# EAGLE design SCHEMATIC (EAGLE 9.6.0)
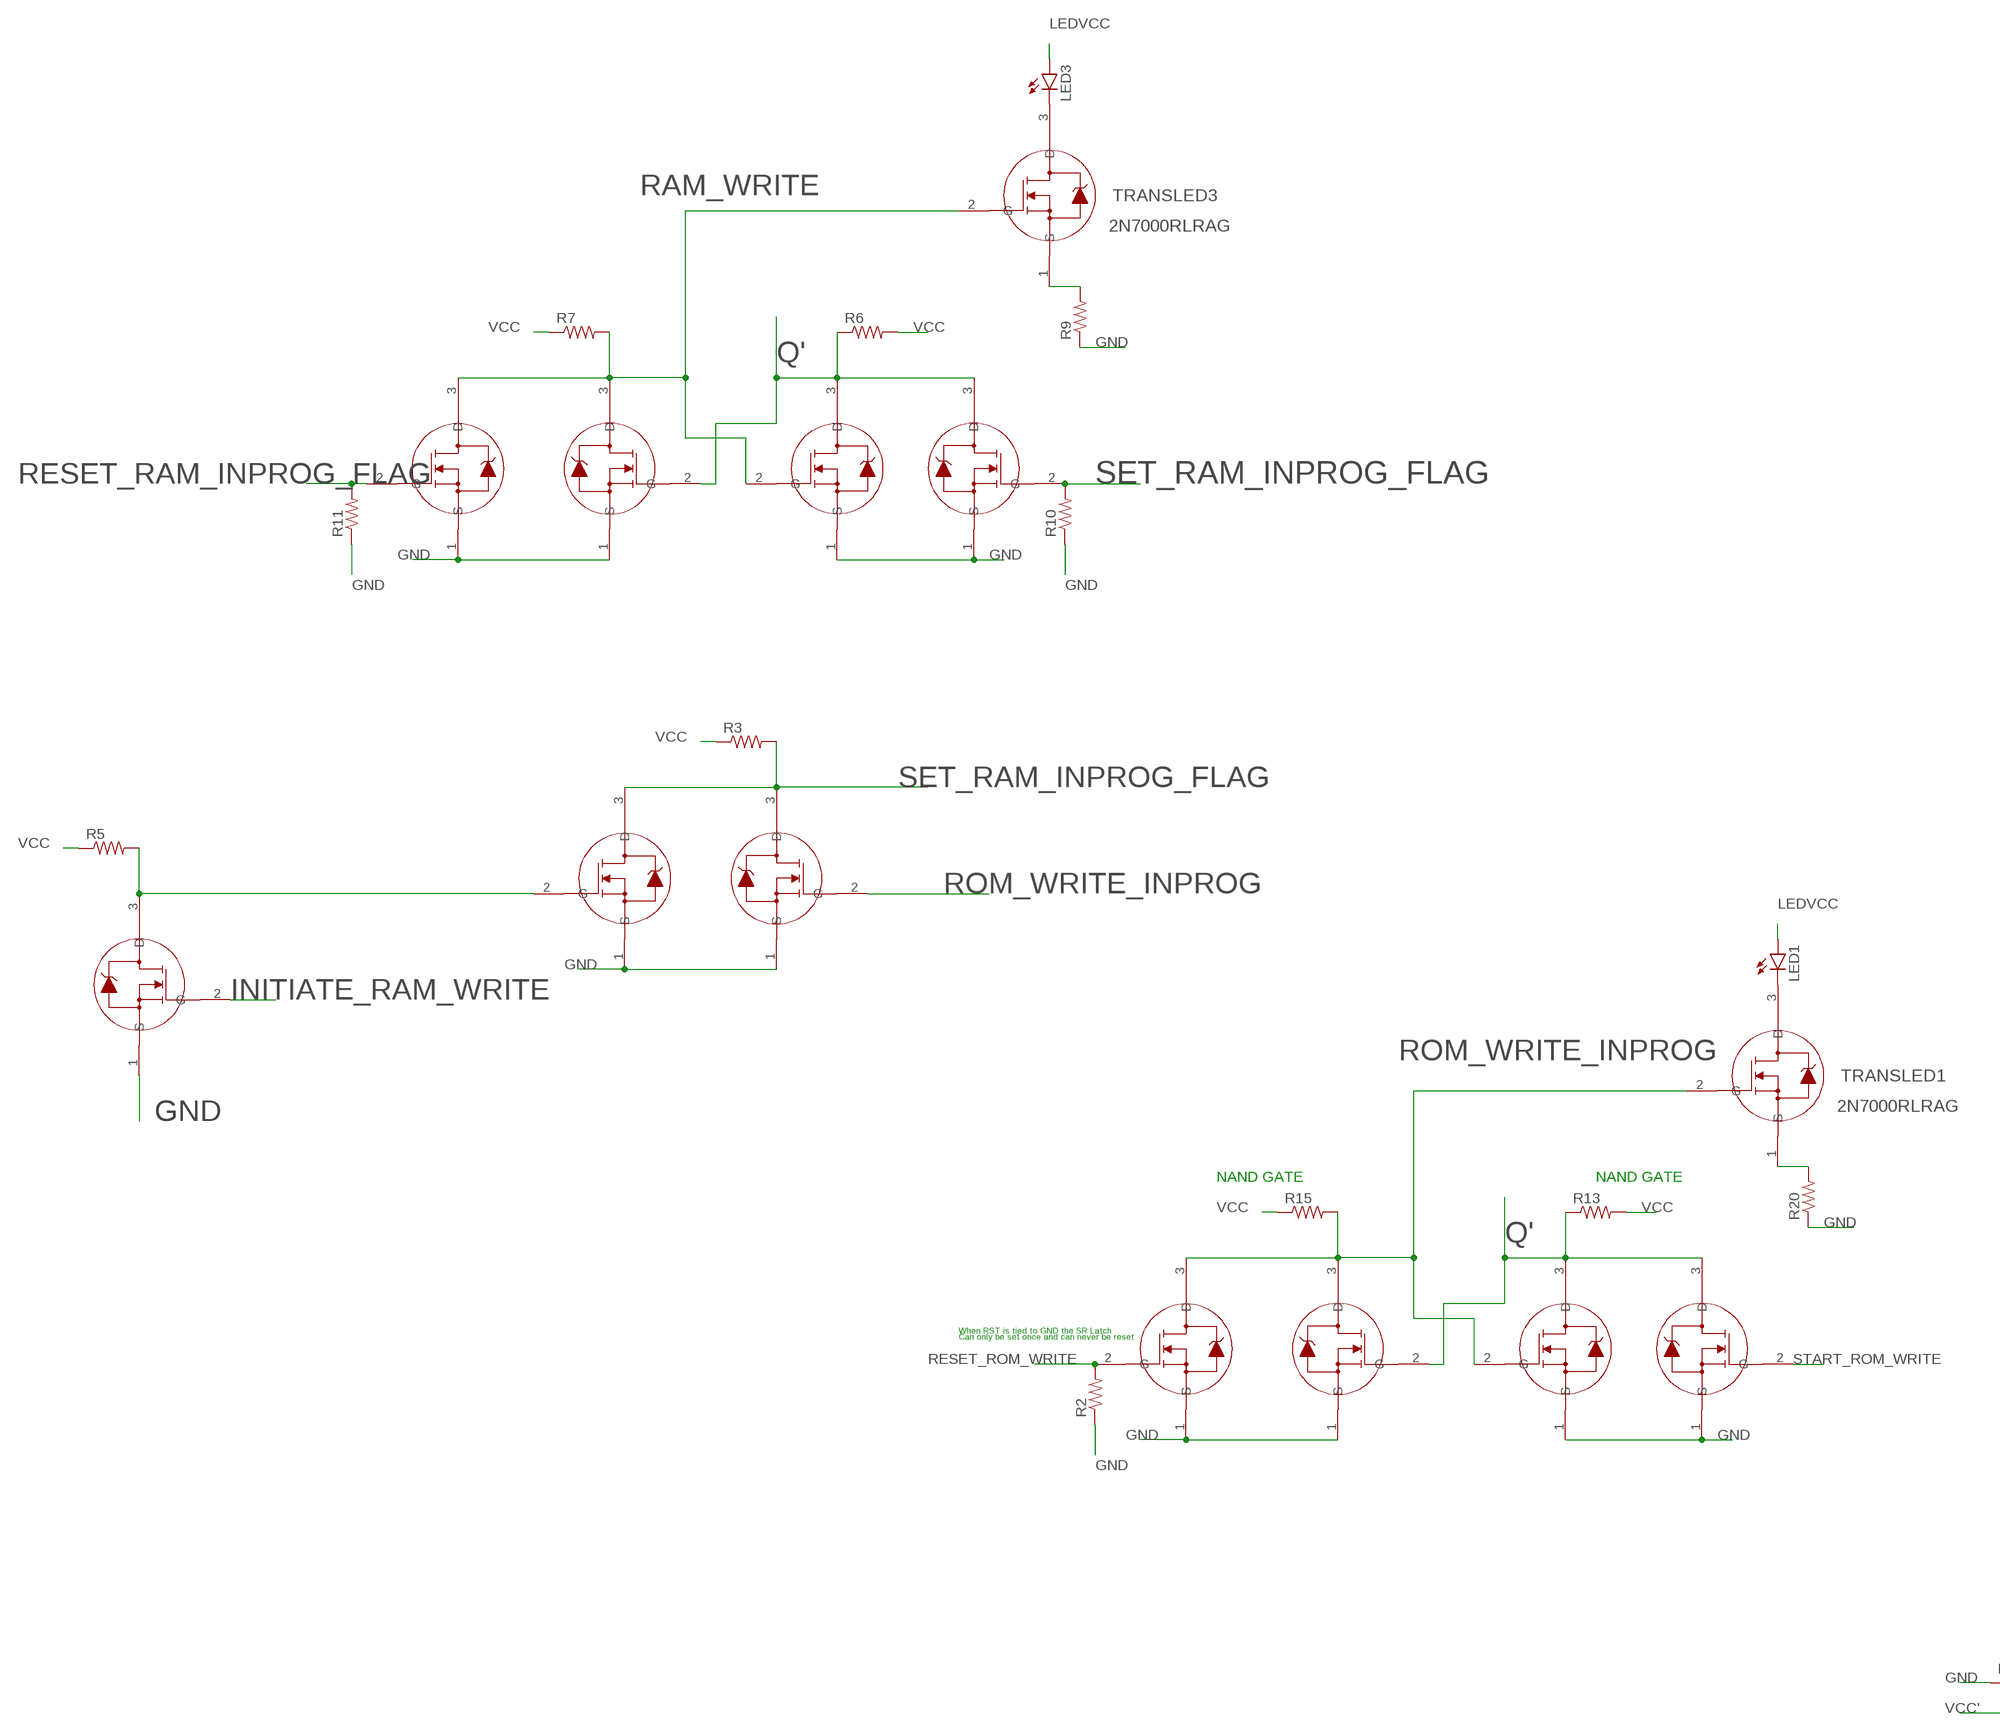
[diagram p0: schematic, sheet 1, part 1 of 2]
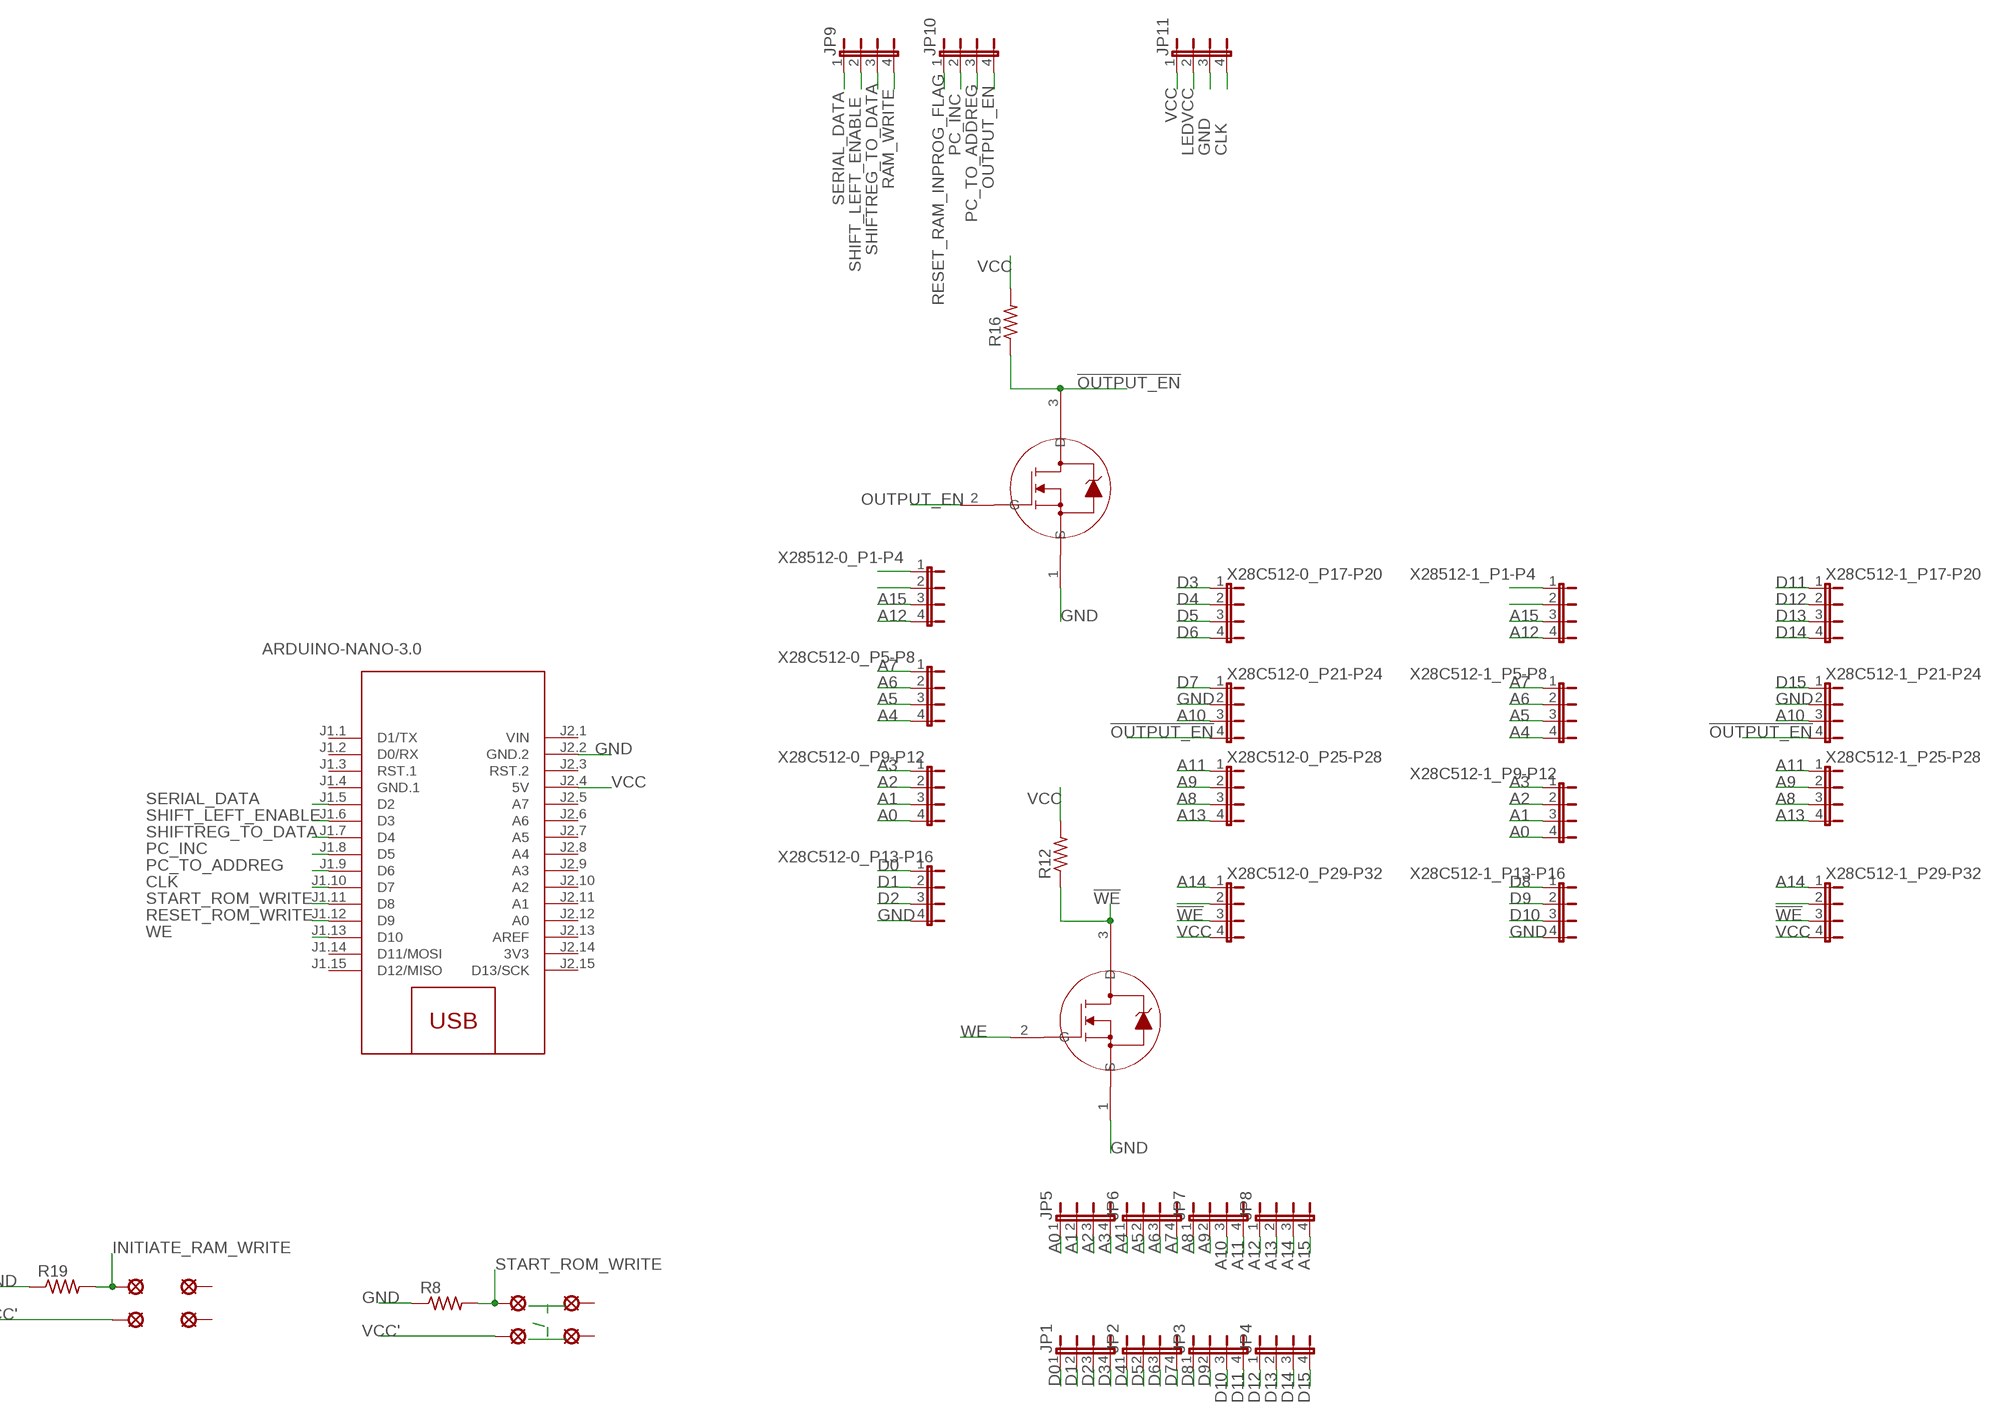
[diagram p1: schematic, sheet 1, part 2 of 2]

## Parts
B1_BL  SE14  [SE14]
B1_BL3  SE14  [SE14]
B1_BR  SE14  [SE14]
B1_BR3  SE14  [SE14]
B1_TL  SE14  [SE14]
B1_TL3  SE14  [SE14]
B1_TR  SE14  [SE14]
B1_TR3  SE14  [SE14]
JP1  JP4E  [JP4]
JP2  JP4E  [JP4]
JP3  JP4E  [JP4]
JP4  JP4E  [JP4]
JP5  JP4E  [JP4]
JP6  JP4E  [JP4]
JP7  JP4E  [JP4]
JP8  JP4E  [JP4]
JP9  JP4E  [JP4]
JP10  JP4E  [JP4]
JP11  JP4E  [JP4]
LED1  LED3MM  [LED3MM]
LED3  LED3MM  [LED3MM]
M1  ARDUINO-NANO-3.0  [ARDUINO-NANO-3.0]
NFET1  2N7000RLRAG  [TO-92_ONS]
NFET2  2N7000RLRAG  [TO-92_ONS]
NFET3  2N7000RLRAG  [TO-92_ONS]
NFET4  2N7000RLRAG  [TO-92_ONS]
NFET5  2N7000RLRAG  [TO-92_ONS]
NFET6  2N7000RLRAG  [TO-92_ONS]
NFET7  2N7000RLRAG  [TO-92_ONS]
NFET8  2N7000RLRAG  [TO-92_ONS]
NFET10  2N7000RLRAG  [TO-92_ONS]
NFET19  2N7000RLRAG  [TO-92_ONS]
NFET20  2N7000RLRAG  [TO-92_ONS]
NFET21  2N7000RLRAG  [TO-92_ONS]
NFET22  2N7000RLRAG  [TO-92_ONS]
R2  R-US_0204/7  [0204/7]
R3  R-US_0204/7  [0204/7]
R5  R-US_0204/7  [0204/7]
R6  R-US_0204/7  [0204/7]
R7  R-US_0204/7  [0204/7]
R8  R-US_0204/7  [0204/7]
R9  R-US_0204/7  [0204/7]
R10  R-US_0204/7  [0204/7]
R11  R-US_0204/7  [0204/7]
R12  R-US_0204/7  [0204/7]
R13  R-US_0204/7  [0204/7]
R15  R-US_0204/7  [0204/7]
R16  R-US_0204/7  [0204/7]
R19  R-US_0204/7  [0204/7]
R20  R-US_0204/7  [0204/7]
TRANSLED1  2N7000RLRAG  [TO-92_ONS]
TRANSLED3  2N7000RLRAG  [TO-92_ONS]
X28C512-0_P5-P8  JP4E  [JP4]
X28C512-0_P9-P12  JP4E  [JP4]
X28C512-0_P13-P16  JP4E  [JP4]
X28C512-0_P17-P20  JP4E  [JP4]
X28C512-0_P21-P24  JP4E  [JP4]
X28C512-0_P25-P28  JP4E  [JP4]
X28C512-0_P29-P32  JP4E  [JP4]
X28C512-1_P5-P8  JP4E  [JP4]
X28C512-1_P9-P12  JP4E  [JP4]
X28C512-1_P13-P16  JP4E  [JP4]
X28C512-1_P17-P20  JP4E  [JP4]
X28C512-1_P21-P24  JP4E  [JP4]
X28C512-1_P25-P28  JP4E  [JP4]
X28C512-1_P29-P32  JP4E  [JP4]
X28512-0_P1-P4  JP4E  [JP4]
X28512-1_P1-P4  JP4E  [JP4]

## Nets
!OUTPUT_EN: NFET10.3(D) R16.1 X28C512-0_P21-P24.4 X28C512-1_P21-P24.4
!WE: NFET4.3(D) R12.1 X28C512-0_P29-P32.3 X28C512-1_P29-P32.3
A0: JP5.1 X28C512-0_P9-P12.4 X28C512-1_P9-P12.4
A1: JP5.2 X28C512-0_P9-P12.3 X28C512-1_P9-P12.3
A2: JP5.3 X28C512-0_P9-P12.2 X28C512-1_P9-P12.2
A3: JP5.4 X28C512-0_P9-P12.1 X28C512-1_P9-P12.1
A4: JP6.1 X28C512-0_P5-P8.4 X28C512-1_P5-P8.4
A5: JP6.2 X28C512-0_P5-P8.3 X28C512-1_P5-P8.3
A6: JP6.3 X28C512-0_P5-P8.2 X28C512-1_P5-P8.2
A7: JP6.4 X28C512-0_P5-P8.1 X28C512-1_P5-P8.1
A8: JP7.1 X28C512-0_P25-P28.3 X28C512-1_P25-P28.3
A9: JP7.2 X28C512-0_P25-P28.2 X28C512-1_P25-P28.2
A10: JP7.3 X28C512-0_P21-P24.3 X28C512-1_P21-P24.3
A11: JP7.4 X28C512-0_P25-P28.1 X28C512-1_P25-P28.1
A12: JP8.1 X28512-0_P1-P4.4 X28512-1_P1-P4.4
A13: JP8.2 X28C512-0_P25-P28.4 X28C512-1_P25-P28.4
A14: JP8.3 X28C512-0_P29-P32.1 X28C512-1_P29-P32.1
A15: JP8.4 X28512-0_P1-P4.3 X28512-1_P1-P4.3
CLK: JP11.4 M1.J1.10(D7)
D0: JP1.1 X28C512-0_P13-P16.1
D1: JP1.2 X28C512-0_P13-P16.2
D2: JP1.3 X28C512-0_P13-P16.3
D3: JP1.4 X28C512-0_P17-P20.1
D4: JP2.1 X28C512-0_P17-P20.2
D5: JP2.2 X28C512-0_P17-P20.3
D6: JP2.3 X28C512-0_P17-P20.4
D7: JP2.4 X28C512-0_P21-P24.1
D8: JP3.1 X28C512-1_P13-P16.1
D9: JP3.2 X28C512-1_P13-P16.2
D10: JP3.3 X28C512-1_P13-P16.3
D11: JP3.4 X28C512-1_P17-P20.1
D12: JP4.1 X28C512-1_P17-P20.2
D13: JP4.2 X28C512-1_P17-P20.3
D14: JP4.3 X28C512-1_P17-P20.4
D15: JP4.4 X28C512-1_P21-P24.1
GND: JP11.3 M1.J2.2(GND.2) NFET1.1(S) NFET2.1(S) NFET3.1(S) NFET4.1(S) NFET5.1(S) NFET6.1(S) NFET7.1(S) NFET8.1(S) NFET10.1(S) NFET19.1(S) NFET20.1(S) NFET21.1(S) NFET22.1(S) R2.1 R8.1 R9.1 R10.1 R11.1 R19.1 R20.1 X28C512-0_P13-P16.4 X28C512-0_P21-P24.2 X28C512-1_P13-P16.4 X28C512-1_P21-P24.2
INITIATE_RAM_WRITE: B1_TL3.MP NFET3.2(G) R19.2
LEDVCC: JP11.2 LED1.A LED3.A
N$1: X28512-0_P1-P4.1
N$2: X28512-0_P1-P4.2
N$5: LED3.K(C) TRANSLED3.3(D)
N$6: R9.2 TRANSLED3.1(S)
N$17: X28512-1_P1-P4.1
N$18: X28512-1_P1-P4.2
N$22: X28C512-0_P29-P32.2
N$41: LED1.K(C) TRANSLED1.3(D)
N$42: R20.2 TRANSLED1.1(S)
N$44: X28C512-1_P29-P32.2
OUTPUT_EN: JP10.4 NFET10.2(G)
PC_INC: JP10.2 M1.J1.8(D5)
PC_TO_ADDREG: JP10.3 M1.J1.9(D6)
Q': NFET5.2(G) NFET7.3(D) NFET8.3(D) NFET19.2(G) NFET21.3(D) NFET22.3(D) R6.1 R13.1
RAM_WRITE: JP9.4 NFET5.3(D) NFET6.3(D) NFET7.2(G) R7.2 TRANSLED3.2(G)
RAM_WRITE_FLAG: NFET2.2(G) NFET3.3(D) R5.2
RESET_RAM_INPROG_FLAG: JP10.1 NFET6.2(G) R11.2
RESET_ROM_WRITE: M1.J1.12(D9) NFET20.2(G) R2.2
ROM_WRITE_INPROG: NFET1.2(G) NFET19.3(D) NFET20.3(D) NFET21.2(G) R15.2 TRANSLED1.2(G)
SERIAL_DATA: JP9.1 M1.J1.5(D2)
SET_RAM_INPROG_FLAG: NFET1.3(D) NFET2.3(D) NFET8.2(G) R3.2 R10.2
SHIFT_LEFT_ENABLE: JP9.2 M1.J1.6(D3)
SHIFTREG_TO_DATA: JP9.3 M1.J1.7(D4)
START_ROM_WRITE: B1_TL.MP M1.J1.11(D8) NFET22.2(G) R8.2
VCC: JP11.1 M1.J2.4(5V) R3.1 R5.1 R6.2 R7.1 R12.2 R13.2 R15.1 R16.2 X28C512-0_P29-P32.4 X28C512-1_P29-P32.4
VCC': B1_BL3.MP B1_BL.MP
WE: M1.J1.13(D10) NFET4.2(G)
Unconnected: B1_BR3.MP B1_BR.MP B1_TR3.MP B1_TR.MP M1.J1.1(D1/TX) M1.J1.2(D0/RX) M1.J1.3(RST.1) M1.J1.14(D11/MOSI) M1.J1.15(D12/MISO) M1.J2.3(RST.2) M1.J2.5(A7) M1.J2.6(A6) M1.J2.7(A5) M1.J2.8(A4) M1.J2.9(A3) M1.J2.10(A2) M1.J2.11(A1) M1.J2.12(A0) M1.J2.13(AREF) M1.J2.15(D13/SCK)

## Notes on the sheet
- NAND GATE | NAND GATE
- Can only be set once and can never be reset | When RST is tied to GND the SR Latch
- ____
- ____ | _ | _/  _

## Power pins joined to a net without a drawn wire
3V3: M1.J2.14(3V3)
GND.1: M1.J1.4(GND.1)
VIN: M1.J2.1(VIN)

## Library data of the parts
B1_BL B1_BL3 B1_BR B1_BR3 B1_TL B1_TL3 B1_TR B1_TR3 = solpad:SE14: SOLDER PAD
JP1-JP11 X28C512-0_P5-P8 X28C512-0_P9-P12 X28C512-0_P13-P16 X28C512-0_P17-P20 X28C512-0_P21-P24 X28C512-0_P25-P28 X28C512-0_P29-P32 X28C512-1_P5-P8 X28C512-1_P9-P12 X28C512-1_P13-P16 X28C512-1_P17-P20 X28C512-1_P21-P24 X28C512-1_P25-P28 X28C512-1_P29-P32 X28512-0_P1-P4 X28512-1_P1-P4 = jumper:JP4E: JUMPER
LED1 LED3 = led:LED: LED
M1 = JD-WEEK_8_9_1:ARDUINO-NANO-3.0: Arduino Nano 3.0 and compatible devices More details available here: https://www.arduino.cc/en/Main/ArduinoBoardNano Click here to find device on ebay.com
NFET1-NFET8 NFET10 NFET19-NFET22 TRANSLED1 TRANSLED3 = Transistor(MOSFET):2N7000RLRAG; COPYRIGHT: Copyright (C) 2022 Ultra Librarian. All rights reserved.; MANUFACTURER_PART_NUMBER: 2N7000RLRAG; MFR_NAME: onsemi
R2 R3 R5-R13 R15 R16 R19 R20 = rcl:R-US_: RESISTOR, American symbol; SPICEPREFIX: R

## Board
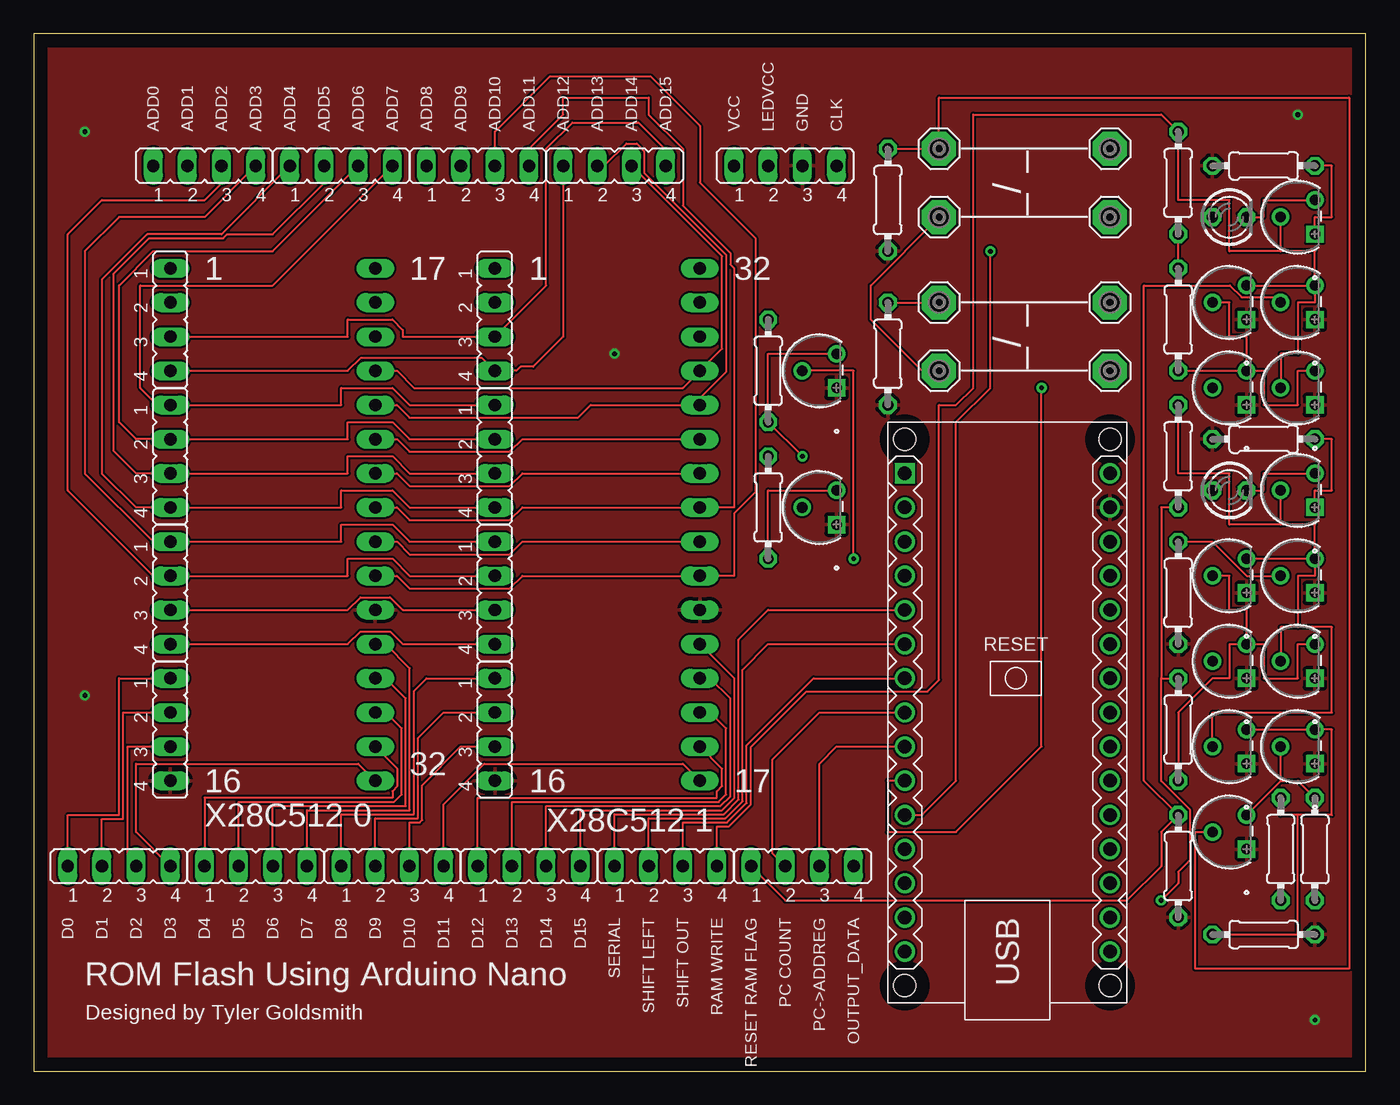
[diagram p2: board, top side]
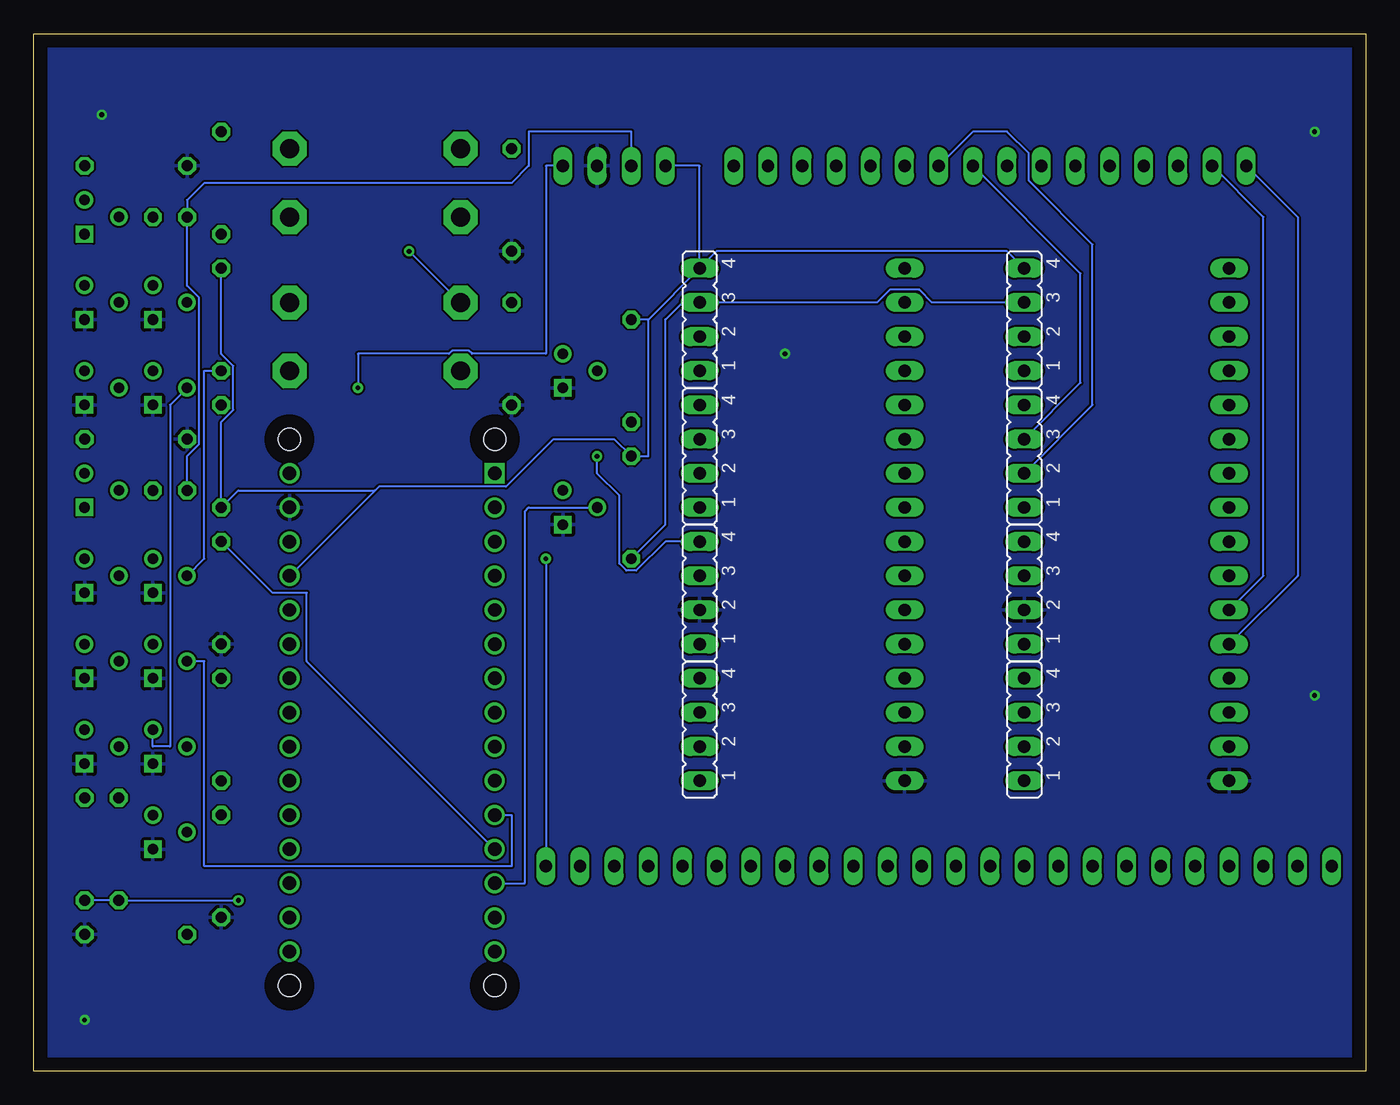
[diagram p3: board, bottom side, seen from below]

Size 99.04 x 77.14 mm. Coordinates in mm from the lower left corner, seen from the top.
Outline: 0,0 99.04,0 99.04,77.14 0,77.14 0,0
Copper layers (1*16): Top 0.035mm / dielectric 1.5mm / Bottom 0.035mm
Design rules "default *": minimum track width 6mil, minimum drill 0.35mm, track to track 6mil, track to pad 6mil, pad to pad 6mil, via to via 6mil, smd to smd 6mil, copper to edge 40mil, drill to drill 6mil, minimum pad ring 10mil, minimum via ring 8mil, stop-mask expansion 4mil, vias tented up to drill 0mil, thermal gap 10mil

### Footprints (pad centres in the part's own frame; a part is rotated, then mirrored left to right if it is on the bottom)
SE14 = drill 1.397 pad 2.54 octagon: MP 0,0
JP4 = drill 0.914 long: 1 -3.81,0; 2 -1.27,0; 3 1.27,0; 4 3.81,0
LED3MM = drill 0.813 octagon: A -1.27,0; K 1.27,0
ARDUINO-NANO-3.0 = drill 1 square: J1.1 17.78,7.62 | drill 1: J1.2 15.24,7.62; J1.3 12.7,7.62; J1.4 10.16,7.62; J1.5 7.62,7.62; J1.6 5.08,7.62; J1.7 2.54,7.62; J1.8 0,7.62; J1.9 -2.54,7.62; J1.10 -5.08,7.62; J1.11 -7.62,7.62; J1.12 -10.16,7.62; J1.13 -12.7,7.62; J1.14 -15.24,7.62; J1.15 -17.78,7.62; J2.1 17.78,-7.62; J2.2 15.24,-7.62; J2.3 12.7,-7.62; J2.4 10.16,-7.62; J2.5 7.62,-7.62; J2.6 5.08,-7.62; J2.7 2.54,-7.62; J2.8 0,-7.62; J2.9 -2.54,-7.62; J2.10 -5.08,-7.62; J2.11 -7.62,-7.62; J2.12 -10.16,-7.62; J2.13 -12.7,-7.62; J2.14 -15.24,-7.62; J2.15 -17.78,-7.62 | hole 1.651: -20.32,7.62; -20.32,-7.62; 20.32,-7.62; 20.32,7.62
TO-92_ONS = drill 0.787 pad 1.295 square: 1 0,0 | drill 0.787 pad 1.295: 2 1.27,2.54; 3 2.54,0
0204/7 = drill 0.813 octagon: 1 -3.81,0; 2 3.81,0

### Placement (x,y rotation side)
B1_BL  67.31,52.07 0 top
B1_BL3  67.31,63.5 0 top
B1_BR  80.01,52.07 0 top
B1_BR3  80.01,63.5 0 top
B1_TL  67.31,57.15 0 top
B1_TL3  67.31,68.58 0 top
B1_TR  80.01,57.15 0 top
B1_TR3  80.01,68.58 0 top
JP1  6.35,15.24 0 top
JP2  16.51,15.24 0 top
JP3  26.67,15.24 0 top
JP4  36.83,15.24 0 top
JP5  12.7,67.31 0 top
JP6  22.86,67.31 0 top
JP7  33.02,67.31 0 top
JP8  43.18,67.31 0 top
JP9  46.99,15.24 0 top
JP10  57.15,15.24 0 top
JP11  55.88,67.31 0 top
LED1  88.9,43.18 0 top
LED3  88.9,63.5 0 top
M1  72.39,26.67 90 top
NFET1  90.17,22.86 90 top
NFET2  95.25,22.86 90 top
NFET3  90.17,16.51 90 top
NFET4  59.69,40.64 90 top
NFET5  90.17,55.88 90 top
NFET6  95.25,55.88 90 top
NFET7  95.25,49.53 90 top
NFET8  90.17,49.53 90 top
NFET10  59.69,50.8 90 top
NFET19  90.17,35.56 90 top
NFET20  95.25,35.56 90 top
NFET21  95.25,29.21 90 top
NFET22  90.17,29.21 90 top
R2  85.09,35.56 90 top
R3  92.71,16.51 90 top
R5  95.25,16.51 90 top
R6  85.09,55.88 90 top
R7  85.09,66.04 90 top
R8  63.5,53.34 90 top
R9  91.44,67.31 0 top
R10  91.44,10.16 180 top
R11  85.09,15.24 90 top
R12  54.61,41.91 90 top
R13  85.09,25.4 90 top
R15  85.09,45.72 90 top
R16  54.61,52.07 90 top
R19  63.5,64.77 90 top
R20  91.44,46.99 0 top
TRANSLED1  95.25,41.91 90 top
TRANSLED3  95.25,62.23 90 top
X28C512-0_P5-P8  10.16,45.72 270 top
X28C512-0_P9-P12  10.16,35.56 270 top
X28C512-0_P13-P16  10.16,25.4 270 top
X28C512-0_P17-P20  25.4,25.4 90 bottom
X28C512-0_P21-P24  25.4,35.56 90 bottom
X28C512-0_P25-P28  25.4,45.72 90 bottom
X28C512-0_P29-P32  25.4,55.88 90 bottom
X28C512-1_P5-P8  34.29,45.72 270 top
X28C512-1_P9-P12  34.29,35.56 270 top
X28C512-1_P13-P16  34.29,25.4 270 top
X28C512-1_P17-P20  49.53,25.4 90 bottom
X28C512-1_P21-P24  49.53,35.56 90 bottom
X28C512-1_P25-P28  49.53,45.72 90 bottom
X28C512-1_P29-P32  49.53,55.88 90 bottom
X28512-0_P1-P4  10.16,55.88 270 top
X28512-1_P1-P4  34.29,55.88 270 top

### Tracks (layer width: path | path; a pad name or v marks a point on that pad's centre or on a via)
!OUTPUT_EN  (via drill 0.35)
  Top 0.152: X28C512-0_P21-P24.4 27.01,39.37 27.95,38.43 35.39,38.43 36.33,39.37 X28C512-1_P21-P24.4 | NFET10.3 54.61,53.34 R16.1 v57.15,45.72
  Bottom 0.152: v57.15,45.72 57.15,44.45 55.5,42.8 55.5,37.73 54.98,37.21 54.24,37.21 52.08,39.37 X28C512-1_P21-P24.4
!WE
  Top 0.152: R12.1 54.61,43.18 NFET4.3
  Bottom 0.152: R12.1 52.07,40.64 52.07,55.88 50.8,57.15 X28C512-1_P29-P32.3 36.33,57.15 35.39,58.09 33.19,58.09 32.25,57.15 X28C512-0_P29-P32.3
A0
  Top 0.152: X28C512-0_P9-P12.4 23.36,31.75 24.3,32.69 26.5,32.69 27.44,31.75 X28C512-1_P9-P12.4
  Bottom 0.152: JP5.1 5.08,63.5 5.08,36.83 X28C512-0_P9-P12.4
A1
  Top 0.152: X28C512-0_P9-P12.3 23.36,34.29 24.3,35.23 26.5,35.23 27.44,34.29 X28C512-1_P9-P12.3
  Bottom 0.152: X28C512-0_P9-P12.3 7.62,36.83 7.62,63.5 JP5.2
A2
  Top 0.152: JP5.3 13.97,66.04 12.7,64.77 5.08,64.77 2.54,62.23 2.54,43.18 8.89,36.83 X28C512-0_P9-P12.2 23.36,36.83 23.36,38.1 26.67,38.1 27.94,36.83 X28C512-1_P9-P12.2
A3
  Top 0.152: JP5.4 12.7,63.5 6.35,63.5 3.81,60.96 3.81,44.45 8.89,39.37 X28C512-0_P9-P12.1 22.86,39.37 22.86,40.64 26.67,40.64 27.94,39.37 X28C512-1_P9-P12.1
A4
  Top 0.152: JP6.1 13.97,62.23 8.46,62.23 5.08,58.85 5.08,44.45 7.62,41.91 X28C512-0_P5-P8.4 22.86,41.91 22.86,43.18 26.67,43.18 27.94,41.91 X28C512-1_P5-P8.4
A5
  Top 0.152: JP6.2 21.59,66.04 17.78,62.23 14.4,62.23 14.1,61.92 8.59,61.92 5.97,59.31 5.97,46.1 7.62,44.45 X28C512-0_P5-P8.3 23.36,44.45 23.36,45.72 26.67,45.72 27.94,44.45 X28C512-1_P5-P8.3
A6
  Top 0.152: JP6.3 17.78,60.96 8.89,60.96 6.35,58.42 6.35,48.26 7.62,46.99 X28C512-0_P5-P8.2 23.36,46.99 23.36,48.26 26.67,48.26 27.94,46.99 X28C512-1_P5-P8.2
A7
  Top 0.152: JP6.4 17.78,58.42 7.92,58.42 7.92,50.8 9.2,49.53 X28C512-0_P5-P8.1 22.86,49.53 22.86,50.8 26.67,50.8 27.94,49.53 X28C512-1_P5-P8.1
A8
  Top 0.152: X28C512-0_P25-P28.3 27.01,46.99 27.95,46.05 35.39,46.05 36.33,46.99 X28C512-1_P25-P28.3
  Bottom 0.152: JP7.1 21.21,59.31 21.21,51.18 X28C512-0_P25-P28.3
A9
  Top 0.152: X28C512-0_P25-P28.2 27.01,44.45 27.95,43.51 35.39,43.51 36.33,44.45 X28C512-1_P25-P28.2
  Bottom 0.152: X28C512-0_P25-P28.2 20.32,49.53 20.32,61.46 25.07,66.21 25.07,68.25 26.67,69.85 29.21,69.85 JP7.2
A10
  Top 0.152: X28C512-0_P21-P24.3 27.01,36.83 27.95,35.89 35.39,35.89 36.33,36.83 X28C512-1_P21-P24.3 52.07,36.83 52.07,41.48 53.64,43.05 53.64,61.95 49.53,66.06 49.53,70.28 45.85,73.97 38.41,73.97 34.29,69.85 JP7.3
A11
  Top 0.152: X28C512-0_P25-P28.1 27.01,41.91 27.95,40.97 35.39,40.97 36.33,41.91 X28C512-1_P25-P28.1 52.07,41.91 52.07,59.69 51.79,59.97 51.79,60.83 48.26,64.36 48.26,68.58 45.72,71.12 45.72,72.39 39.37,72.39 39.37,71.12 36.83,68.58 JP7.4
A12
  Top 0.152: X28512-0_P1-P4.4 23.36,52.07 24.3,53.01 33.35,53.01 X28512-1_P1-P4.4 35.9,52.07 36.2,52.38 37.14,52.38 39.37,54.61 JP8.1
A13
  Top 0.152: X28C512-0_P25-P28.4 27.01,49.53 27.95,48.59 40.47,48.59 41.41,49.53 X28C512-1_P25-P28.4 49.53,50.03 51.49,51.99 51.49,60.7 45.39,66.8 45.39,68.41 44.84,68.96 44.06,68.96 42.41,67.31 JP8.2
A14
  Top 0.152: X28C512-0_P29-P32.1 27.01,52.07 28.28,50.8 48.26,50.8 X28C512-1_P29-P32.1 51.18,53.72 51.18,60.58 JP8.3
A15
  Top 0.152: X28512-0_P1-P4.3 23.36,54.61 23.36,55.88 26.67,55.88 27.44,55.11 27.44,54.61 X28512-1_P1-P4.3 38.1,58.42 38.1,68.58 40.06,70.54 44.97,70.54 46.99,68.51 JP8.4
CLK  (via drill 0.35)
  Top 0.152: M1.J1.10 63.5,21.59 63.5,17.78 68.58,17.78 74.93,24.13 v74.93,50.8
  Bottom 0.152: JP11.4 60.96,67.31 60.96,53.34 66.46,53.34 66.69,53.57 67.93,53.57 68.16,53.34 74.93,53.34 v74.93,50.8
D0
  Top 0.152: JP1.1 2.54,19.05 6.35,19.05 6.35,29.21 X28C512-0_P13-P16.1
D1
  Top 0.152: JP1.2 5.08,18.74 6.66,18.74 6.66,26.67 X28C512-0_P13-P16.2
D2
  Top 0.152: JP1.3 6.96,15.9 6.96,24.13 X28C512-0_P13-P16.3
D3
  Top 0.152: JP1.4 7.62,17.78 7.62,22.86 24.13,22.86 X28C512-0_P17-P20.1
D4
  Top 0.152: X28C512-0_P17-P20.2 27.05,22.48 27.05,21.2 26.67,20.82 26.67,20.32 12.7,20.32 JP2.1
D5
  Top 0.152: JP2.2 15.24,20.02 26.8,20.02 27.36,20.58 27.36,25.48 26.17,26.67 X28C512-0_P17-P20.3
D6
  Top 0.152: JP2.3 17.78,19.71 27.66,19.71 27.66,27.72 26.17,29.21 X28C512-0_P17-P20.4
D7
  Top 0.152: JP2.4 20.32,19.41 27.97,19.41 27.97,29.95 26.17,31.75 X28C512-0_P21-P24.1
D8
  Top 0.152: JP3.1 22.86,19.1 28.27,19.1 28.27,28.27 29.21,29.21 X28C512-1_P13-P16.1
D9
  Top 0.152: JP3.2 25.4,18.8 28.57,18.8 28.58,18.8 28.58,24.77 30.48,26.67 X28C512-1_P13-P16.2
D10
  Top 0.152: JP3.3 27.94,18.49 28.7,18.49 28.88,18.67 28.88,21.26 31.75,24.13 X28C512-1_P13-P16.3
D11
  Top 0.152: JP3.4 30.48,19.84 33.5,22.86 48.26,22.86 X28C512-1_P17-P20.1
D12
  Top 0.152: JP4.1 33.02,20.32 50.8,20.32 50.8,20.82 51.18,21.2 51.18,22.48 X28C512-1_P17-P20.2
D13
  Top 0.152: JP4.2 35.56,20.02 50.93,20.02 51.49,20.58 51.49,25.48 50.3,26.67 X28C512-1_P17-P20.3
D14
  Top 0.152: JP4.3 38.1,19.71 51.05,19.71 51.79,20.45 51.79,27.72 50.3,29.21 X28C512-1_P17-P20.4
D15
  Top 0.152: JP4.4 40.64,19.41 51.18,19.41 52.09,20.32 52.09,29.19 X28C512-1_P21-P24.1
GND  (via drill 0.35)
  other vias: 3.81,69.85 93.98,71.12 95.25,3.81 3.81,27.94 43.18,53.34
  pour Top: -10.16,80.01 101.6,80.01 101.6,-2.54 -8.89,-2.54 -10.16,-1.27
  pour Bottom: -10.16,80.01 101.6,80.01 101.6,-2.54 -8.89,-2.54 -10.16,-1.27
INITIATE_RAM_WRITE
  Top 0.152: R19.2 B1_TL3.MP 67.31,72.39 97.79,72.39 97.79,7.62 86.36,7.62 86.36,17.78 NFET3.2
LEDVCC
  Bottom 0.152: JP11.2 54.61,69.85 62.23,69.85 62.23,67.31 63.5,66.04 86.36,66.04 87.63,64.77 LED3.A 87.63,58.39 86.74,57.5 86.74,46.62 87.63,45.73 LED1.A
N$5
  Top 0.152: LED3.K 91.44,63.5 91.44,64.77 TRANSLED3.3
N$6
  Top 0.152: TRANSLED3.1 95.25,63.5 96.52,63.5 96.52,67.31 R9.2
N$41
  Top 0.152: LED1.K 91.44,43.18 91.44,44.45 TRANSLED1.3
N$42
  Top 0.152: TRANSLED1.1 95.25,43.18 96.52,43.18 96.52,46.99 R20.2
OUTPUT_EN  (via drill 0.35)
  Top 0.152: v60.96,38.1 60.96,52.07 NFET10.2
  Bottom 0.152: v60.96,38.1 JP10.4
PC_INC
  Top 0.152: JP10.2 54.89,16.23 54.89,23.14 58.42,26.67 M1.J1.8
PC_TO_ADDREG
  Top 0.152: JP10.3 58.42,22.86 59.69,24.13 M1.J1.9
Q'
  Top 0.152: NFET22.3 91.44,31.75 91.44,29.21 93.98,29.21 93.98,31.75 NFET21.3 | NFET22.3 88.9,31.75 88.9,29.21 87.63,29.21 85.09,26.67 R13.1 | NFET22.3 90.17,34.29 88.9,34.29 88.9,36.83 NFET19.2 | NFET8.3 91.44,52.07 91.44,49.53 93.98,49.53 93.98,52.07 NFET7.3 | R6.1 NFET8.3 | NFET8.3 90.17,54.61 88.9,54.61 88.9,57.15 NFET5.2
  Bottom 0.152: NFET19.2 86.36,38.1 86.36,52.07 R6.1
RAM_WRITE
  Top 0.152: NFET6.3 95.25,60.96 92.71,60.96 | 92.71,60.96 TRANSLED3.2 | NFET5.3 NFET6.3 | NFET6.3 95.25,57.15 93.98,57.15 93.98,53.34 92.71,53.34 NFET7.2 | 92.71,60.96 88.9,60.96 88.9,64.77 85.09,64.77 R7.2 83.82,71.12 69.85,71.12 69.85,50.8 68.58,49.53 67.31,49.53 67.31,29.09 66.45,28.23 57.44,28.23 53.31,24.11 53.31,19.82 51.68,18.19 50.8,18.19 JP9.4
RAM_WRITE_FLAG
  Top 0.152: NFET3.3 92.71,21.59 | 92.71,21.59 NFET2.2 | 92.71,21.59 93.98,21.59 R5.2
RESET_RAM_INPROG_FLAG
  Top 0.152: NFET6.2 92.32,57.54 89.81,57.54 88.93,58.42 82.55,58.42 82.55,21.59 R11.2 83.82,17.78 83.82,15.24 81.28,12.7 55.88,12.7 JP10.1
RESET_ROM_WRITE
  Top 0.152: R2.2 87.63,39.37 90.17,36.83 NFET20.2
  Bottom 0.152: M1.J1.12 78.74,30.48 78.74,35.56 81.28,35.56 R2.2
ROM_WRITE_INPROG
  Top 0.152: NFET20.3 95.25,40.64 92.71,40.64 | 92.71,40.64 TRANSLED1.2 | NFET19.3 NFET20.3 | NFET20.3 95.25,36.83 93.98,36.83 93.98,33.02 | 93.98,33.02 92.71,33.02 NFET21.2 | 92.71,40.64 88.9,40.64 88.9,44.45 85.09,44.45 R15.2 | 93.98,33.02 96.52,33.02 96.52,26.67 87.63,26.67 NFET1.2
SERIAL_DATA
  Top 0.152: JP9.1 43.18,19.1 51.3,19.1 52.4,20.2 52.4,32.08 54.61,34.29 M1.J1.5
SET_RAM_INPROG_FLAG
  Top 0.152: R3.2 92.71,19.05 93.98,19.05 | 93.98,19.05 96.52,19.05 96.52,25.4 NFET2.3 NFET1.3 | R10.2 93.98,10.16 93.98,19.05
  Bottom 0.152: NFET8.2 88.9,49.53 88.9,24.13 90.17,24.13 NFET1.3
SHIFT_LEFT_ENABLE
  Top 0.152: JP9.2 45.72,18.8 51.43,18.8 52.7,20.07 52.7,29.84 54.61,31.75 M1.J1.6
SHIFTREG_TO_DATA
  Top 0.152: JP9.3 48.26,18.49 51.56,18.49 53.01,19.94 53.01,24.23 57.99,29.21 M1.J1.7
START_ROM_WRITE  (via drill 0.35)
  Top 0.152: R8.2 B1_TL.MP | M1.J1.11 66.04,19.05 68.58,21.59 68.58,48.26 71.12,50.8 v71.12,60.96
  Bottom 0.152: M1.J1.11 63.5,19.05 63.5,15.24 86.36,15.24 86.36,30.48 NFET22.2 | B1_TL.MP v71.12,60.96
VCC  (via drill 0.35)
  Top 0.152: R6.2 R7.1 | R15.1 83.82,41.91 83.82,29.21 | 83.82,29.21 R13.2 | v83.82,12.7 85.09,13.97 85.09,14.81 85.98,15.7 85.98,19.42 83.82,21.58 83.82,29.21
  Bottom 0.152: X28C512-0_P29-P32.4 26.67,60.96 48.26,60.96 X28C512-1_P29-P32.4 | X28C512-1_P29-P32.4 49.53,67.31 JP11.1 | X28C512-1_P29-P32.4 53.34,55.88 | 53.34,55.88 R16.2 | 53.34,55.88 53.34,45.72 R12.2 55.88,46.99 60.4,46.99 63.92,43.47 73.37,43.47 73.66,43.18 | 73.66,43.18 M1.J2.4 | R6.2 85.09,53.33 84.2,52.44 84.2,49.16 85.09,48.27 R15.1 83.82,43.18 73.66,43.18 | R5.1 R3.1 v83.82,12.7
VCC'
  Top 0.152: B1_BL.MP 66.04,52.07 62.23,55.88 62.23,58.42 B1_BL3.MP
WE
  Bottom 0.152: M1.J1.13 62.52,13.97 62.52,41.62 62.23,41.91 NFET4.2

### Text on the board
tNames: ADD0 | ADD1 | ADD2 | ADD3 | ADD4 | ADD5 | ADD6 | ADD7 | ADD8 | ADD9 | ADD10 | ADD11 | ADD12 | ADD13 | ADD14 | ADD15 | VCC | LEDVCC | GND | CLK | _______ | _/ _ | _______ | 1 | 17 | 1 | 32 | _______ | _/ _ | _______ | 32 | 16 | 16 | 17 | X28C512 0 | X28C512 1 | D0 | D1 | D2 | D3 | D4 | D5 | D6 | D7 | D8 | D9 | D10 | D11 | D12 | D13 | D14 | D15 | SERIAL | SHIFT LEFT | SHIFT OUT | RAM WRITE | RESET RAM FLAG | PC COUNT | PC->ADDREG | OUTPUT_DATA | ROM Flash Using Arduino Nano | Designed by Tyler Goldsmith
